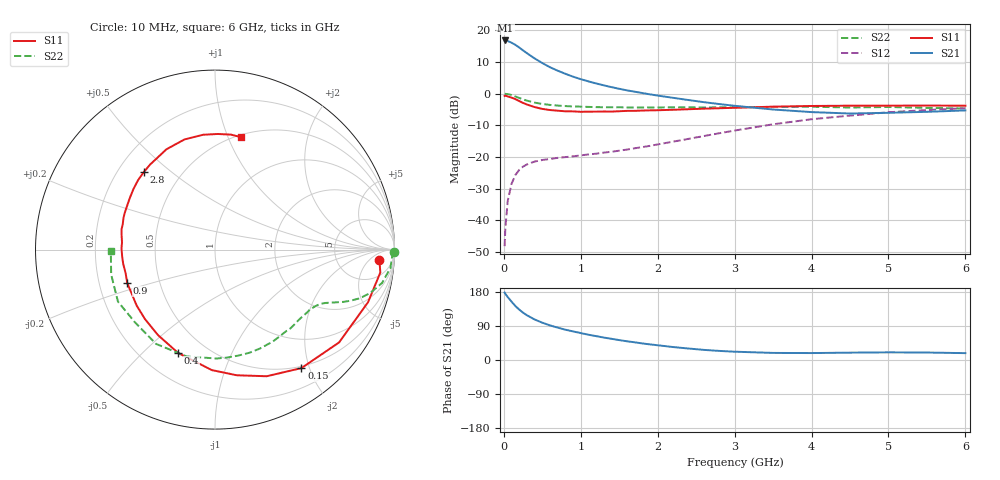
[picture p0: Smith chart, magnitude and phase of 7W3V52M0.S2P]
! Infineon Technologies  Discrete & RF Semiconductors
! BFS17W
! Si NPN RF Bipolar Junction Transistor in SOT323
! VCE = 3.5 V  IC = 2 mA
! Common Emitter S-Parameters:  August  1999
# GHz  S  MA  R  50
!  f  S11  S21  S12  S22
! GHz  MAG  ANG  MAG  ANG  MAG  ANG  MAG  ANG
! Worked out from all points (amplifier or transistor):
!   36 points, 10 MHz to 6 GHz, reference 50 ohm
!   highest |S21| = 16.8 dB at 20 MHz (marker M1)
!   |S21| within 3 dB of that: start of sweep to 242.6 MHz
!   unconditionally stable (mu >= 1): 823.6 MHz to 3.432 GHz; 3.659 GHz to end of sweep
!   at 250 MHz: K = 0.36, MSG = 18.3 dB, |S12| = -23.1 dB
!   at 1.4 GHz: K = 1.31, MAG = 6.9 dB, |S12| = -18.4 dB
!   at 6 GHz: K = 1.09, MAG = -2.2 dB, |S12| = -4.6 dB
!   S11 on the Smith chart (normalised r, x): 10 MHz: 15, -11; 150 MHz: 0.47, -1.87; 400 MHz: 0.35, -0.65; 900 MHz: 0.32, -0.17; 2.8 GHz: 0.31, +0.40; 6 GHz: 0.52, +1.12
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0.01  0.9182 -3.7  6.869 177.9  0.0039 89.3  0.9993 -0.7
0.02  0.9299 -7.9  6.89 174.6  0.0076 85.0  0.9877 -2.3
0.05  0.9016 -19.0  6.742 166.3  0.02 79.2  0.9826 -6.0
0.1  0.8634 -36.8  6.353 154.1  0.0376 70.4  0.9491 -11.3
0.15  0.8171 -53.9  5.873 142.4  0.0518 61.4  0.8994 -15.5
0.2  0.7621 -67.8  5.328 133.0  0.0624 56.3  0.8528 -18.5
0.25  0.7105 -80.2  4.803 124.9  0.0703 50.6  0.8084 -20.6
0.3  0.6716 -91.5  4.34 118.1  0.0761 47.4  0.7736 -22.1
0.4  0.6115 -109.6  3.588 106.9  0.0845 42.2  0.7196 -24.2
0.5  0.5725 -123.7  3.03 98.5  0.0894 40.1  0.6851 -25.7
0.6  0.5497 -135.2  2.603 91.3  0.0928 39.4  0.6621 -27.1
0.7  0.5364 -144.4  2.296 85.4  0.0966 39.7  0.6464 -28.8
0.9  0.5234 -159.2  1.847 75.4  0.1021 41.6  0.6252 -32.4
1.1  0.5175 -171.1  1.557 66.7  0.1094 44.6  0.6155 -36.6
1.3  0.521 179.2  1.348 59.2  0.117 47.7  0.6081 -41.4
1.6  0.5328 167.7  1.123 49.4  0.1306 53.0  0.6031 -48.8
2.2  0.5546 149.0  0.856 34.2  0.1741 61.4  0.6055 -65.5
2.8  0.5862 132.7  0.683 24.0  0.2362 63.9  0.6053 -83.5
3.5  0.621 115.8  0.56 18.7  0.3271 60.7  0.6159 -104.9
4.5  0.6433 95.9  0.484 19.4  0.4486 48.9  0.6025 -137.7
5.5  0.6467 82.1  0.515 19.7  0.5491 36.1  0.595 -166.4
6  0.6428 76.9  0.542 18.1  0.5878 30.0  0.5807 -179.0
